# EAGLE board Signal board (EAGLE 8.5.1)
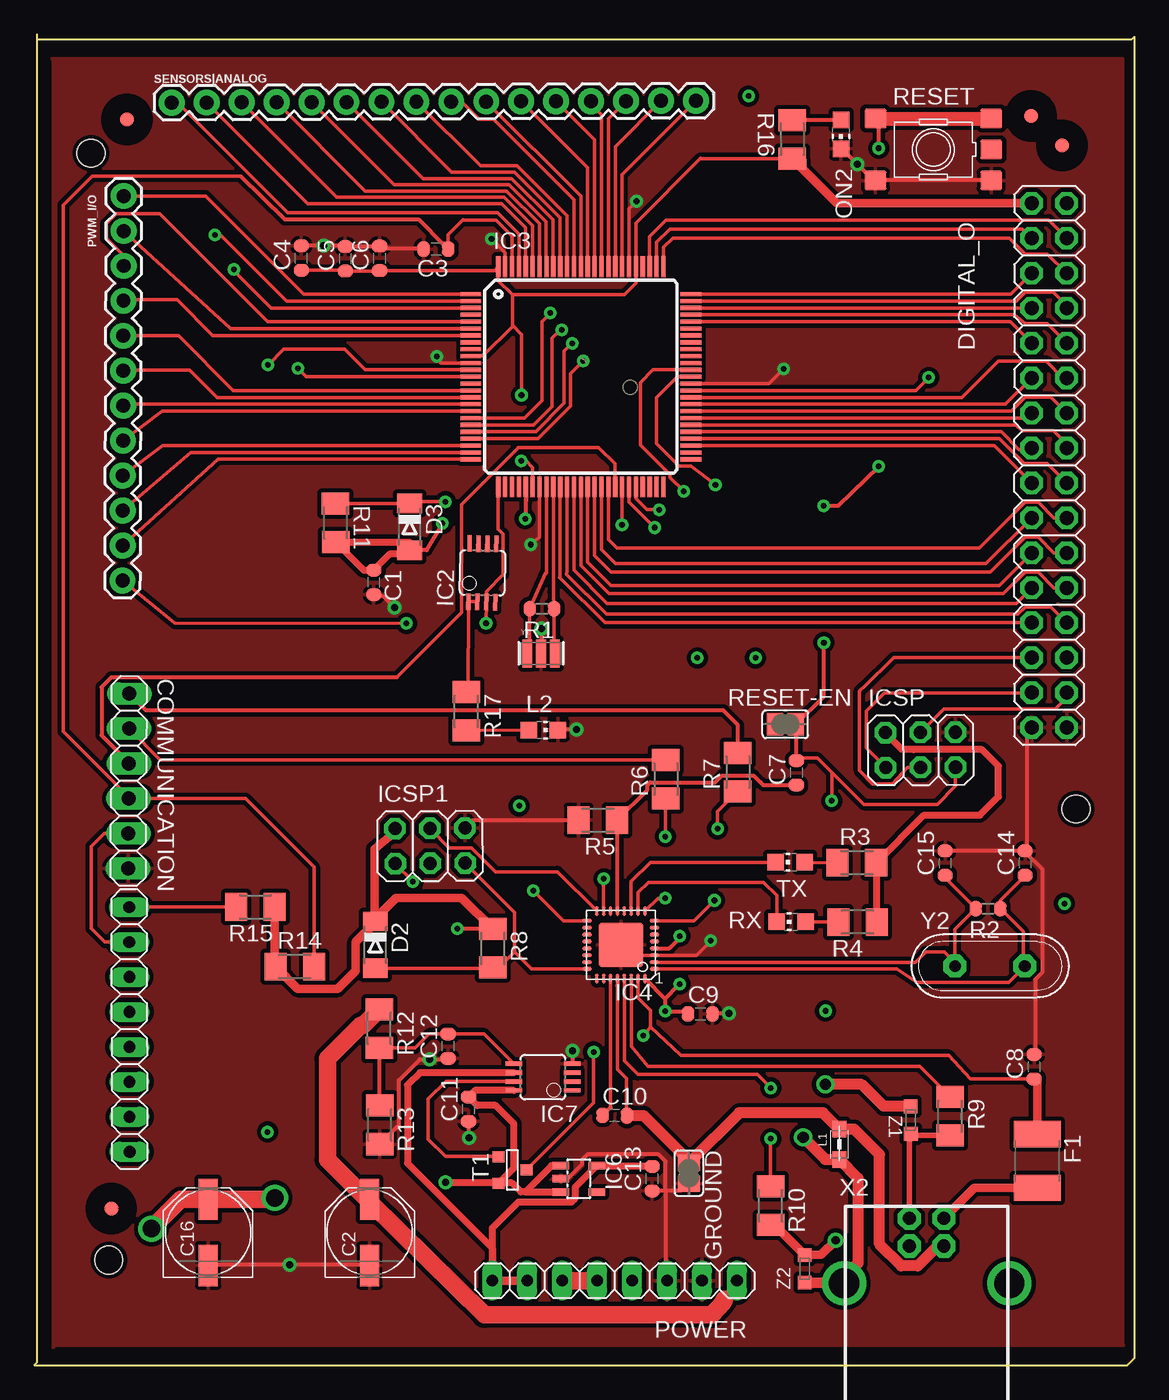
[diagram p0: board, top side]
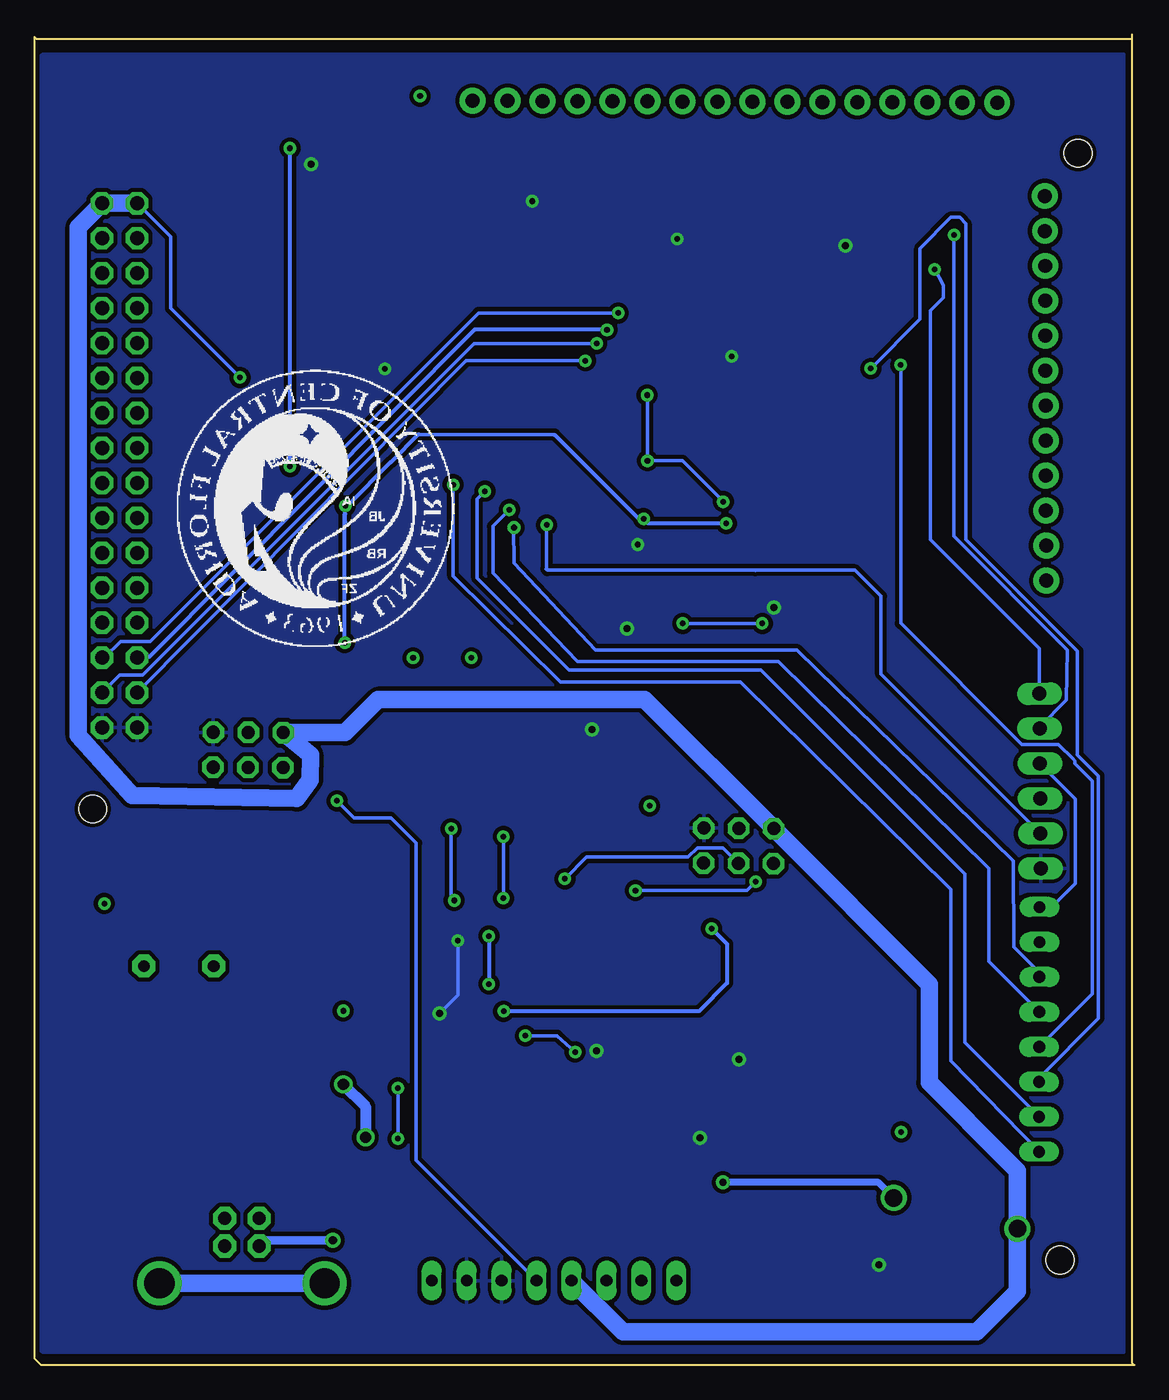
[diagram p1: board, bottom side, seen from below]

Size 79.92 x 96.68 mm. Coordinates in mm from the lower left corner, seen from the top.
Outline: 0.17,96.34 79.75,96.34 79.92,96.51 79.92,0.51 79.41,0 0,0 0.17,0.17 0.17,96.68
Copper layers (1*16): Top 0.035mm / dielectric 1.5mm / Bottom 0.035mm
Design rules "SparkFun *": minimum track width 8mil, minimum drill 8mil, track to track 8mil, track to pad 8mil, pad to pad 8mil, via to via 8mil, smd to smd 8mil, copper to edge 8mil, drill to drill 8mil, minimum pad ring 12mil, minimum via ring 10mil, stop-mask expansion 4mil, vias tented up to drill 20mil, thermal gap 10mil
Net classes: 0 default: width 0.203 mm, drill 0.406 mm, clearance 0.203 mm; 1 power: width 0.61 mm, drill 0.406 mm, clearance 0.203 mm; 2 gnd: width 0.305 mm, drill 0.406 mm, clearance 0.203 mm; 3 power usb: width 0.508 mm, drill 0.406 mm, clearance 0.203 mm
Holes 2.03 mm at 5.4,7.64 75.68,40.4 4.1,88.05

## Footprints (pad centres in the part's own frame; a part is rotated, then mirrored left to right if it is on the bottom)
C0603-ROUND = smd 0.898 x 1.1: 1 -0.889,0; 2 0.889,0
PANASONIC_D = smd 3 x 1.4: + 2.4,0; - -2.4,0
1X08 = drill 0.85 pad 1.422 long: 1 -8.89,0; 2 -6.35,0; 3 -3.81,0; 4 -1.27,0; 5 1.27,0; 6 3.81,0; 7 6.35,0; 8 8.89,0
MINIMELF = smd 1.4 x 1.8: A 1.7,0; C -1.7,0
2X16 = drill 1.016 octagon: 1 -19.05,-1.27; 2 -19.05,1.27; 3 -16.51,-1.27; 4 -16.51,1.27; 5 -13.97,-1.27; 6 -13.97,1.27; 7 -11.43,-1.27; 8 -11.43,1.27; 9 -8.89,-1.27; 10 -8.89,1.27; 11 -6.35,-1.27; 12 -6.35,1.27; 13 -3.81,-1.27; 14 -3.81,1.27; 15 -1.27,-1.27; 16 -1.27,1.27; 17 1.27,-1.27; 18 1.27,1.27; 19 3.81,-1.27; 20 3.81,1.27; 21 6.35,-1.27; 22 6.35,1.27; 23 8.89,-1.27; 24 8.89,1.27; 25 11.43,-1.27; 26 11.43,1.27; 27 13.97,-1.27; 28 13.97,1.27; 29 16.51,-1.27; 30 16.51,1.27; 31 19.05,-1.27; 32 19.05,1.27
L1812 = smd 1.9 x 3.4: 1 -1.95,0; 2 1.95,0
FIDUCIA-MOUNT = smd 1.016 x 1.016: P$1 0,0
SJ = smd 1.168 x 1.6: 1 -0.762,0; 2 0.762,0
MSOP08 = smd 0.3 x 1.2: 1 -0.976,-2.113; 2 -0.326,-2.113; 3 0.324,-2.113; 4 0.974,-2.113; 5 0.974,2.112; 6 0.324,2.112; 7 -0.326,2.112; 8 -0.976,2.112
TQFP100 = smd 1.5 x 0.3: 1 -8,6; 2 -8,5.5; 3 -8,5; 4 -8,4.5; 5 -8,4; 6 -8,3.5; 7 -8,3; 8 -8,2.5; 9 -8,2; 10 -8,1.5; 11 -8,1; 12 -8,0.5; 13 -8,0; 14 -8,-0.5; 15 -8,-1; 16 -8,-1.5; 17 -8,-2; 18 -8,-2.5; 19 -8,-3; 20 -8,-3.5; 21 -8,-4; 22 -8,-4.5; 23 -8,-5; 24 -8,-5.5; 25 -8,-6; 51 8,-6; 52 8,-5.5; 53 8,-5; 54 8,-4.5; 55 8,-4; 56 8,-3.5; 57 8,-3; 58 8,-2.5; 59 8,-2; 60 8,-1.5; 61 8,-1; 62 8,-0.5; 63 8,0; 64 8,0.5; 65 8,1; 66 8,1.5; 67 8,2; 68 8,2.5; 69 8,3; 70 8,3.5; 71 8,4; 72 8,4.5; 73 8,5; 74 8,5.5; 75 8,6 | smd 0.3 x 1.5: 26 -6,-8; 27 -5.5,-8; 28 -5,-8; 29 -4.5,-8; 30 -4,-8; 31 -3.5,-8; 32 -3,-8; 33 -2.5,-8; 34 -2,-8; 35 -1.5,-8; 36 -1,-8; 37 -0.5,-8; 38 0,-8; 39 0.5,-8; 40 1,-8; 41 1.5,-8; 42 2,-8; 43 2.5,-8; 44 3,-8; 45 3.5,-8; 46 4,-8; 47 4.5,-8; 48 5,-8; 49 5.5,-8; 50 6,-8; 76 6,8; 77 5.5,8; 78 5,8; 79 4.5,8; 80 4,8; 81 3.5,8; 82 3,8; 83 2.5,8; 84 2,8; 85 1.5,8; 86 1,8; 87 0.5,8; 88 0,8; 89 -0.5,8; 90 -1,8; 91 -1.5,8; 92 -2,8; 93 -2.5,8; 94 -3,8; 95 -3.5,8; 96 -4,8; 97 -4.5,8; 98 -5,8; 99 -5.5,8; 100 -6,8
MLF32 = smd 0.7 x 0.28: 1 -2.45,1.75; 2 -2.45,1.25; 3 -2.45,0.75; 4 -2.45,0.25; 5 -2.45,-0.25; 6 -2.45,-0.75; 7 -2.45,-1.25; 8 -2.45,-1.75; 17 2.45,-1.75; 18 2.45,-1.25; 19 2.45,-0.75; 20 2.45,-0.25; 21 2.45,0.25; 22 2.45,0.75; 23 2.45,1.25; 24 2.45,1.75 | smd 0.28 x 0.7: 9 -1.75,-2.45; 10 -1.25,-2.45; 11 -0.75,-2.45; 12 -0.25,-2.45; 13 0.25,-2.45; 14 0.75,-2.45; 15 1.25,-2.45; 16 1.75,-2.45; 25 1.75,2.45; 26 1.25,2.45; 27 0.75,2.45; 28 0.25,2.45; 29 -0.25,2.45; 30 -0.75,2.45; 31 -1.25,2.45; 32 -1.75,2.45 | smd 3.254 x 3.254: 33 0,0
SOT23-DBV = smd 0.55 x 1.2: 1 -0.95,-1.3; 2 0,-1.3; 3 0.95,-1.3; 4 0.95,1.3; 5 -0.95,1.3
2X03 = drill 0.95 pad 1.55 octagon: 1 -2.54,-1.27; 2 -2.54,1.27; 3 0,-1.27; 4 0,1.27; 5 2.54,-1.27; 6 2.54,1.27
0805 = smd 1.2 x 1: 1 -1.1,0; 2 1.1,0
CHIP-LED0805 = smd 1.2 x 1.2: A 0,-1.05; C 0,1.05
1X12 = drill 1.016 pad 1.88: 1 0,0; 2 2.54,0; 3 5.08,0; 4 7.62,0; 5 10.16,0; 6 12.7,0; 7 15.24,0; 8 17.78,0; 9 20.32,0; 10 22.86,0; 11 25.4,0; 12 27.94,0
R0603-ROUND = smd 0.898 x 1.1: 1 -0.889,0; 2 0.889,0
M1206 = smd 1.6 x 2: 1 -1.4,0; 2 1.4,0
TS42 = smd 1.6 x 1.4: 1 -4.2,2.25; 2 4.2,2.25; 3 -4.2,-2.25; 4 4.2,-2.25; 5 -4.2,0
1X16 = drill 1.016 pad 1.88: 1 0,0; 2 2.54,0; 3 5.08,0; 4 7.62,0; 5 10.16,0; 6 12.7,0; 7 15.24,0; 8 17.78,0; 9 20.32,0; 10 22.86,0; 11 25.4,0; 12 27.94,0; 13 30.48,0; 14 33.02,0; 15 35.56,0; 16 38.1,0
SOT-23 = smd 0.787 x 0.889: 1 0.025,-1.016; 2 -0.94,1.016; 3 0.991,1.016
PN61729 = drill 0.95 pad 1.676 octagon: 1 1.25,4.71; 2 -1.25,4.71; 3 -1.25,2.71; 4 1.25,2.71 | drill 2.2: P$1 -6,0; P$2 6,0
RESONATOR = smd 0.7 x 2: 1 -1,0; 2 0,0; 3 1,0
QS = drill 0.85 pad 1.676 octagon: 1 -2.54,0; 2 2.54,0
CT/CN0603 = smd 1 x 1: 1 -1,0; 2 1,0
1X06 = drill 1.016 long: 1 -6.35,0; 2 -3.81,0; 3 -1.27,0; 4 1.27,0; 5 3.81,0; 6 6.35,0

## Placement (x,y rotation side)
C1  22p  [C0603-ROUND]  24.66,56.87 270 top
C2  [PANASONIC_D]  24.36,9.64 90 top
C3  100n  [C0603-ROUND]  29.18,81.08 180 top
C4  100n  [C0603-ROUND]  19.39,80.43 90 top
C5  100n  [C0603-ROUND]  22.59,80.38 90 top
C6  100n  [C0603-ROUND]  25.09,80.42 90 top
C7  100n  [C0603-ROUND]  55.37,43.03 90 top
C8  100n  [C0603-ROUND]  72.64,21.67 90 top
C9  100n  [C0603-ROUND]  48.38,25.51 0 top
C10  1u  [C0603-ROUND]  42.17,18.14 0 top
C11  100n  [C0603-ROUND]  31.55,18.6 90 top
C12  100n  [C0603-ROUND]  30.06,23.17 90 top
C13  1u  [C0603-ROUND]  44.88,13.54 90 top
C14  22p  [C0603-ROUND]  71.99,36.48 90 top
C15  22p  [C0603-ROUND]  66.17,36.47 90 top
C16  [PANASONIC_D]  12.62,9.64 90 top
COMMUNICATION  [1X08]  6.9,24.39 270.1 top
D2  CD1206-S01575  [MINIMELF]  24.78,30.53 270 top
D3  CD1206-S01575  [MINIMELF]  27.27,60.9 270 top
DIGITAL_O  [2X16]  73.73,65.36 270 top
F1  MF-MSMF050-2 500mA  [L1812]  72.88,14.83 270 top
FD1  FIDUCIALMOUNT  [FIDUCIA-MOUNT]  6.74,90.51 0 top
FD2  FIDUCIALMOUNT  [FIDUCIA-MOUNT]  72.41,90.77 0 top
FD3  FIDUCIALMOUNT  [FIDUCIA-MOUNT]  5.58,11.39 0 top
FD4  FIDUCIALMOUNT  [FIDUCIA-MOUNT]  74.65,88.61 0 top
GROUND  [SJ]  47.55,13.94 270 top
IC2  LMV358IDGKR  [MSOP08]  32.55,57.57 358.9 top
IC3  ATMEGA2560-16AU  [TQFP100]  39.7,71.81 0 top
IC4  ATMEGA16U2-MU  [MLF32]  42.61,30.53 180 top
IC6  LP2985-33DBVR  [SOT23-DBV]  39.55,13.54 270 top
IC7  LMV358IDGKR  [MSOP08]  36.95,20.92 90 top
ICSP  [2X03]  64.39,44.69 0.3 top
ICSP1  [2X03]  28.75,37.72 0.4 top
L1  BLM21  [0805]  58.49,16.04 270 top
L2  YELLOW  [CHIP-LED0805]  36.98,46.14 270 top
ON2  GREEN  [CHIP-LED0805]  58.6,89.41 180 top
POWER  [1X08]  42.16,6.14 0 top
PWM_I/O  [1X12]  6.5,84.94 269.8 top
R1  1M  [R0603-ROUND]  36.88,54.94 180 top
R2  1M  [R0603-ROUND]  69.28,33.16 180 top
R3  1k  [M1206]  59.76,36.49 0 top
R4  1k  [M1206]  59.81,32.19 0 top
R5  1k  [M1206]  40.93,39.6 180 top
R6  1k  [M1206]  45.88,42.58 90 top
R7  1k  [M1206]  51.11,43.08 90 top
R8  10k  [M1206]  33.31,30.28 270 top
R9  22R  [M1206]  66.53,18.08 270 top
R10  22R  [M1206]  53.48,11.58 270 top
R11  10k  [M1206]  21.88,61.19 270.4 top
R12  10k  [M1206]  25.06,24.45 270 top
R13  10k  [M1206]  25.09,17.46 270 top
R14  10k  [M1206]  18.91,28.95 0 top
R15  10k  [M1206]  16.06,33.29 180 top
R16  1k  [M1206]  55.07,89.06 90.3 top
R17  1k  [M1206]  31.38,47.49 270 top
RESET  TS42031-160R-TR-7260  [TS42]  65.32,88.32 180 top
RESET-EN  [SJ]  54.56,46.56 0 top
RX  YELLOW  [CHIP-LED0805]  54.99,32.21 90 top
SENSORS|ANALOG  [1X16]  9.97,91.72 0.2 top
T1  FDN340P  [SOT-23]  34.74,14.15 90 top
TX  YELLOW  [CHIP-LED0805]  54.9,36.53 90 top
X2  USB-B_TH  [PN61729]  64.83,5.94 0 top
Y1  CSTCE16M0V53-R0 16MHZ  [RESONATOR]  36.81,51.7 0 top
Y2  16MHz  [QS]  69.43,28.99 0 top
Z1  CG0603MLC-05E  [CT/CN0603]  63.67,17.8 270.5 top
Z2  CG0603MLC-05E  [CT/CN0603]  55.96,7 90 top
|  [1X06]  6.85,42.43 269.6 top

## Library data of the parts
C1 C3-C15 COMMUNICATION FD1-FD4 IC3 IC4 IC6 ICSP ICSP1 POWER R1 R2 RESET X2 Y1 Y2 = SmartPrj
C2 C16 = rcl; SPICEPREFIX: C
D2 D3 = diode
DIGITAL_O | = pinhead
F1 = rcl
GROUND RESET-EN = jumper
IC2 IC7 = linear
L1 = wuerth-elektronik
L2 ON2 RX TX = led
PWM_I/O SENSORS|ANALOG = SparkFun-Connectors
R3-R17 = rcl; SPICEPREFIX: R
T1 = zetex; OC_FARNELL: unknown; OC_NEWARK: unknown
Z1 Z2 = varistor

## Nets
5-GND: RESET.5
+3V3 [power]: C13.2 IC6.5 IC7.6 POWER.1 POWER.2
+5V [power usb]: C4.1 C5.1 C6.1 C9.1 C11.2 C16.+ D2.C D3.C DIGITAL_O.1 DIGITAL_O.2 IC3.10 IC3.31 IC3.61 IC3.80 IC3.100 IC4.4 IC4.32 IC6.1 IC6.3 IC7.8 ICSP1.2 ICSP.2 POWER.3 POWER.4 R3.2 R4.2 R8.1 R11.1 R14.1 R15.1 R16.1 T1.2
ADC0: IC3.97 SENSORS|ANALOG.1
ADC1: IC3.96 SENSORS|ANALOG.2
ADC2: IC3.95 SENSORS|ANALOG.3
ADC3: IC3.94 SENSORS|ANALOG.4
ADC4: IC3.93 SENSORS|ANALOG.5
ADC5: IC3.92 SENSORS|ANALOG.6
ADC6: IC3.91 SENSORS|ANALOG.7
ADC7: IC3.90 SENSORS|ANALOG.8
ADC8: IC3.89 SENSORS|ANALOG.9
ADC9: IC3.88 SENSORS|ANALOG.10
ADC10: IC3.87 SENSORS|ANALOG.11
ADC11: IC3.86 SENSORS|ANALOG.12
ADC12: IC3.85 SENSORS|ANALOG.13
ADC13: IC3.84 SENSORS|ANALOG.14
ADC14: IC3.83 SENSORS|ANALOG.15
ADC15: IC3.82 SENSORS|ANALOG.16
AREF: C3.1 IC3.98 R14.2 |.4
CMP: C12.2 IC7.5 R12.2 R13.1
D+: R10.2 X2.3 Z2.2
D-: R9.2 X2.2 Z1.2
DTR: C7.1 IC4.13 R5.1
GATE_CMD: IC7.7 T1.3
GND [gnd]: C1.2 C2.- C3.2 C4.2 C5.2 C6.2 C8.2 C9.2 C11.1 C12.1 C13.1 C14.2 C15.2 C16.- DIGITAL_O.31 DIGITAL_O.32 GROUND.2 IC3.11 IC3.32 IC3.62 IC3.81 IC3.99 IC4.3 IC4.33 IC6.2 IC7.4 ICSP1.6 ICSP.6 L2.C ON2.C POWER.6 POWER.7 R5.2 R13.2 RESET.1 RESET.2 Y1.2 |.6
L13: IC2.1 IC2.2 R17.1
M8RXD: IC4.9 R6.1
M8TXD: IC4.8 R7.1
MISO2: IC4.17 ICSP1.1
MOSI2: IC4.16 ICSP1.4
N$10: L2.A R17.2
N$11: ON2.A R16.2
N$54: R4.1 RX.A
N$55: R3.1 TX.A
PA0: DIGITAL_O.4 IC3.78
PA1: DIGITAL_O.3 IC3.77
PA2: DIGITAL_O.6 IC3.76
PA3: DIGITAL_O.5 IC3.75
PA4: DIGITAL_O.8 IC3.74
PA5: DIGITAL_O.7 IC3.73
PA6: DIGITAL_O.10 IC3.72
PA7: DIGITAL_O.9 IC3.71
PB0: DIGITAL_O.28 IC3.19
PB1: DIGITAL_O.27 IC3.20 ICSP.3
PB2: DIGITAL_O.30 IC3.21 ICSP.4
PB3: DIGITAL_O.29 IC3.22 ICSP.1
PB4: IC3.23 PWM_I/O.9
PB5: IC3.24 PWM_I/O.10
PB6: IC3.25 PWM_I/O.11
PB7: IC2.3 IC3.26 PWM_I/O.12
PC0: DIGITAL_O.17 IC3.53
PC1: DIGITAL_O.18 IC3.54
PC2: DIGITAL_O.15 IC3.55
PC3: DIGITAL_O.16 IC3.56
PC4: DIGITAL_O.13 IC3.57
PC5: DIGITAL_O.14 IC3.58
PC6: DIGITAL_O.11 IC3.59
PC7: DIGITAL_O.12 IC3.60
PE0: IC3.2 R6.2 |.2
PE1: IC3.3 R7.2 |.1
PE3: IC3.5 PWM_I/O.3
PE4: IC3.6 PWM_I/O.2
PE5: IC3.7 PWM_I/O.4
PG5: IC3.1 PWM_I/O.1
PH3: IC3.15 PWM_I/O.5
PH4: IC3.16 PWM_I/O.6
PH5: IC3.17 PWM_I/O.7
PH6: IC3.18 PWM_I/O.8
PL0: DIGITAL_O.25 IC3.35
PL1: DIGITAL_O.26 IC3.36
PL2: DIGITAL_O.23 IC3.37
PL3: DIGITAL_O.24 IC3.38
PL4: DIGITAL_O.21 IC3.39
PL5: DIGITAL_O.22 IC3.40
PL6: DIGITAL_O.19 IC3.41
PL7: DIGITAL_O.20 IC3.42
RD+: IC4.29 R10.1
RD-: IC4.30 R9.1
RESET: C1.1 C7.2 D3.A IC3.30 ICSP.5 POWER.5 R11.2 RESET-EN.1 RESET-EN.2 RESET.3 RESET.4
RESET2: D2.A IC4.24 ICSP1.5 R8.2
RXD1: COMMUNICATION.3 IC3.45
RXD2: COMMUNICATION.5 IC3.12
RXD3: COMMUNICATION.8 IC3.63
RXL: IC4.10 RX.C
SCK2: IC4.15 ICSP1.3
SCL: COMMUNICATION.1 IC3.43 R15.2 |.3
SDA: COMMUNICATION.2 IC3.44 |.5
TXD1: COMMUNICATION.4 IC3.46
TXD2: COMMUNICATION.6 IC3.13
TXD3: COMMUNICATION.7 IC3.64
TXL: IC4.11 TX.C
UGND [gnd]: C10.2 GROUND.1 IC4.28 L1.1 X2.4
USBVCC [power usb]: C8.1 F1.1 IC4.31 T1.1
USHIELD [gnd]: L1.2 X2.P$1 X2.P$2 Z1.1 Z2.1
V+: IC2.8
V-: IC2.4
VIN [power]: C2.+ R12.1
VUCAP: C10.1 IC4.27
XT1: C14.1 IC4.1 R2.1 Y2.2
XT2: C15.1 IC4.2 R2.2 Y2.1
XTAL1: IC3.34 R1.1 Y1.3
XTAL2: IC3.33 R1.2 Y1.1
XVCC [power usb]: F1.2 X2.1

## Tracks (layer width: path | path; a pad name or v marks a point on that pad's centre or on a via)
+3V3
  Top 0.508: C13.2 40.9,14.43 IC6.5 39.3,12.94 39.3,12.12 39.03,11.85 35.16,11.85 33.27,9.96 POWER.1 33.27,8.49 27.1,14.66 27.1,20.34 28,21.25 IC7.6
  Top 0.61: POWER.1 POWER.2
+5V  (via drill 0.41, 0.51, 1.27)
  Top 0.254: 25.08,79.52 C6.1 | C4.1 22.59,79.54 | C5.1 25.05,79.49 C6.1 | R16.1 48.43,87.66 48.41,87.68 43.7,82.98 IC3.80 43.7,78.6 42.87,77.77 34.72,77.77 | IC3.61 64.03,70.81 v64.98,71.76 | v35.37,65.71 35.71,65.71 36.2,65.21 IC3.31 | 34.72,77.77 33.7,78.79 IC3.100 33.51,79.53 C6.1 | IC3.10 31.72,73.33 32.59,73.33 34.72,75.46 34.72,75.55 | 34.72,75.55 34.72,77.77 | v35.4,70.47 35.4,74.87 34.72,75.55 | v29.86,62.73 27.14,62.73 27.02,62.6 D3.C 22.99,62.6 R11.1
  Top 0.305: R8.1 30.76,31.68 v30.72,31.72 | C9.1 47.3,25.71 v45.82,25.71 45.82,26.62 | IC4.32 45.82,26.62 | 45.82,26.62 46.88,27.68 v46.89,27.68 | IC4.4 46.13,30.28 46.9,31.05 v46.9,31.17
  Top 0.508: R4.2 61.62,31.77 61.62,31.56 61.16,32.02 R3.2 64.63,39.96 68.7,39.96 70.05,41.31 70.05,43.52 68.85,44.72 63.87,44.72 63.87,44.73 63.03,44.73 61.84,45.91 ICSP.2 | 34.01,13.22 34.7,13.22 35.34,12.59 35.67,12.59 | 34.01,13.22 33.73,13.22 T1.2 34.84,14.33 34.84,17.54 33.52,18.87 32.16,18.87 C11.2 32.01,19.95 IC7.8 | 35.67,12.59 IC6.3 | v29.89,13.28 33.97,13.27 34.01,13.22 | IC6.1 37.57,14.49 35.67,12.59
  Top 0.61: ICSP1.2 26.19,38.75 24.7,37.49 24.71,32.32 | D2.C 24.71,32.32 | 22.59,79.54 C5.1 | DIGITAL_O.1 58.32,84.41 R16.1 | 24.71,32.32 24.71,32.39 26.28,33.96 31.04,33.96 R8.1 | 24.71,32.32 24.71,32.1 23.35,30.74 23.35,28.64 22.04,27.34 19.12,27.34 R14.1 17.46,29.01 R15.1
  Top 1.27: POWER.3 POWER.4 | v8.5,9.9 10.64,12.04 C16.+ 17.36,12.04 v17.47,12.15
  Bottom 0.254: 72.31,84.41 DIGITAL_O.2 | v64.98,71.76 70.02,76.79 70.02,81.97 DIGITAL_O.1 | v35.4,70.47 35.37,70.45 v35.37,65.71 32.82,65.71 29.86,62.75 v29.86,62.73
  Bottom 0.305: v30.72,31.72 29.59,30.6 29.59,27.75 31.64,25.71 v45.82,25.71 | v46.9,31.17 v46.9,27.69 v46.89,27.68
  Bottom 0.508: v17.47,12.15 18.59,13.27 v29.89,13.28
  Bottom 1.27: 76.73,82.62 76.73,45.74 72.82,41.39 60.85,41.17 59.87,42.52 59.86,44.34 ICSP.2 57.34,45.95 54.94,48.35 35.58,48.35 ICSP1.2 14.89,27.67 14.89,20.53 9.22,14.85 8.5,14.13 v8.5,9.9 8.5,5.36 11.45,2.41 37.16,2.41 POWER.4 | 76.73,82.62 76.61,82.74 | 76.73,82.62 76.73,82.68 DIGITAL_O.2 DIGITAL_O.1
ADC0
  Top 0.254: IC3.97 35.2,82.15 35.21,82.16 33.64,83.74 18.39,83.73 10.35,91.78 SENSORS|ANALOG.1
ADC1
  Top 0.254: IC3.96 35.68,79.83 35.68,82.63 33.93,84.38 19.86,84.38 SENSORS|ANALOG.2
ADC2
  Top 0.254: IC3.95 36.18,79.83 36.18,82.77 34.12,84.84 21.95,84.84 SENSORS|ANALOG.3
ADC3
  Top 0.254: IC3.94 36.68,79.83 36.68,82.92 34.31,85.3 24.04,85.3 SENSORS|ANALOG.4
ADC4
  Top 0.254: IC3.93 37.18,79.83 37.18,83.07 34.49,85.76 26.13,85.76 SENSORS|ANALOG.5
ADC5
  Top 0.254: IC3.92 37.68,79.83 37.68,83.21 34.68,86.21 28.22,86.21 SENSORS|ANALOG.6
ADC6
  Top 0.254: IC3.91 38.18,79.83 38.18,83.36 34.87,86.67 30.32,86.67 SENSORS|ANALOG.7
ADC7
  Top 0.254: IC3.90 38.68,79.83 38.68,83.51 35.06,87.13 32.41,87.13 SENSORS|ANALOG.8
ADC8
  Top 0.254: SENSORS|ANALOG.9 31.04,91.8 32.3,90.53 33.36,90.53 39.2,84.68 IC3.89
ADC9
  Top 0.254: SENSORS|ANALOG.10 39.7,84.93 IC3.88
ADC10
  Top 0.254: SENSORS|ANALOG.11 40.2,86.98 IC3.87
ADC11
  Top 0.254: SENSORS|ANALOG.12 40.7,89.03 IC3.86
ADC12
  Top 0.254: IC3.85 41.2,90.85 40.45,91.6 SENSORS|ANALOG.13
ADC13
  Top 0.254: IC3.84 41.7,90.55 SENSORS|ANALOG.14
ADC14
  Top 0.254: IC3.83 42.2,88.52 SENSORS|ANALOG.15
ADC15
  Top 0.254: IC3.82 42.7,86.49 SENSORS|ANALOG.16
AREF
  Top 0.254: IC3.98 34.7,82.03 33.54,83.19 31.15,83.19 31.14,83.2 30.06,82.13 C3.1 | 30.36,81.37 30.24,81.25 | |.4 6.96,41.16 | 6.96,41.16 15.34,41.16 20.31,36.19 R14.2 | 15,86.37 4.18,86.37 2.1,84.29 2.1,46.03 6.96,41.16
  Top 0.305: 29.74,81.5 29.74,81.4 | 29.74,81.4 C3.1 30.24,81.25 30.37,81.38 | 29.74,81.4 27.89,83.25 18.19,83.25 15,86.37 | 6.46,41.16 |.4
CMP
  Top 0.254: IC7.5 32.68,24.06 C12.2 28.68,24.06 27.65,23.03 25.1,23.03 25.06,22.99
  Top 0.305: R12.2 25.06,22.99 25.06,19.19 R13.1
D+  (via drill 0.61)
  Top 0.61: v58.23,9.07 57.16,8 Z2.2 53.78,10.18 R10.2
  Bottom 0.61: v58.23,9.07 63.17,9.07 X2.3
D-
  Top 0.203: Z1.2 63.73,16.81 63.58,16.8
  Top 0.406: X2.2 63.58,16.8 Z1.2 | Z1.2 | Z1.2 63.68,16.68 R9.2
DTR
  Top 0.305: IC4.13 42.36,39.6 R5.1 44.53,41.79 44.53,42.13 44.74,42.34 49.46,42.34 49.97,42.84 52.26,42.84 52.76,42.34 52.95,42.14 C7.1
GATE_CMD
  Top 0.254: 33.49,20.62 33.68,20.62 | 33.68,20.62 IC7.7 | 33.69,15.21 T1.3 33.72,15.17 33.7,15.19 33.67,15.16 29.87,15.16 28.61,16.42 28.61,19.33 29.9,20.62 33.68,20.62
GND  (via drill 0.41, 0.51)
  Top 0.254: IC4.33 43.36,29.78 IC4.3 48.1,29.78 v49.15,30.82 | IC3.32 36.7,60.16 v36.07,59.61 | IC3.11 29.54,72.81 v29.25,73.27 | IC3.99 34.2,80.84 v33.21,81.83 | IC3.81 43.2,84.02 v43.74,84.56 | IC3.62 53.38,71.31 v54.45,72.38
  Top 0.305: 48.63,5.9 POWER.7 | C15.2 66.21,37.35 71.9,37.35 C14.2 | C8.2 72.71,22.62 72.71,28.01 73.22,28.51 73.22,36.03 72,37.25 C14.2 | C16.- 12.67,7.28 v18.56,7.28 24.35,7.28 C2.- | ON2.C 58.69,88.36 v59.81,87.24 61.03,86.02 RESET.2 61.23,86.12 69.46,86.12 RESET.1 | C12.1 30.04,22.22 v28.72,22.22 28.01,22.22 26.48,20.69 26.48,17.44 25.16,16.12 R13.2 | 45.89,12.67 47.01,12.67 47.52,13.17 GROUND.2 | 45.89,12.67 45.86,12.67 | 45.86,12.67 44.94,12.67 C13.1 | 45.86,12.67 45.86,14.8 45.35,15.31 40.2,15.31 39.79,14.9 39.79,14.6 38.78,13.58 38.27,13.58 IC6.2 | C4.2 19.47,81.35 v21,81.35 22.52,81.35 C5.2 22.62,81.25 25.06,81.25 C6.2 25.16,81.14 28.21,81.14 C3.2 | v31.56,16.53 31.56,17.64 C11.1 | v50.46,25.57 49.34,25.57 C9.2 | v26.18,55.03 25.37,55.85 C1.2 | v39.08,22.83 39.08,21.91 IC7.4 | v39.39,46.19 38.07,46.19 L2.C | R5.2 39.49,39.59 31.87,39.59 31.36,39.08 ICSP1.6 | v36.85,53.51 36.85,51.78 Y1.2 | 45.89,12.67 45.89,6.16 POWER.6 | C14.2 72.1,37.46 72.1,45.99 72.41,46.29 DIGITAL_O.31
  Bottom 0.254: v50.46,25.57 49.15,26.89 v49.15,30.82
  pour Bottom (isolate 0.305): 0.85,0.93 79.32,0.93 79.41,1.02 79.41,95.16 79.32,95.24 0.76,95.24 0.76,0.93
  pour Top (isolate 0.305): 1.27,94.9 79.07,94.9 79.07,1.52 79.16,1.44 1.52,1.44 1.35,1.27 1.35,94.82
L13
  Top 0.254: R17.1 31.52,48.69 IC2.1 IC2.2
M8RXD  (via drill 0.41)
  Top 0.254: v45.85,38.4 45.85,41.14 R6.1 | IC4.9 45.29,33.91 v45.85,33.91
  Bottom 0.254: v45.85,33.91 v45.85,38.4
M8TXD  (via drill 0.41)
  Top 0.254: IC4.8 47.93,32.28 v49.41,33.76 | v49.64,38.96 49.64,40.21 R7.1
  Bottom 0.254: v49.41,33.76 49.64,33.98 v49.64,38.96
MISO2  (via drill 0.41)
  Top 0.254: IC4.17 38.44,32.28 v36.25,34.48 | v27.5,35.12 26.21,36.41 ICSP1.1
  Bottom 0.254: v36.25,34.48 28.15,34.48 v27.5,35.12
MOSI2
  Top 0.254: 28.77,39.16 ICSP1.4 30.15,37.58 31.76,37.58 33.51,35.83 38,35.83 IC4.16
N$2  (via drill 0.41)
  other vias: 35.22,40.64
N$4  (via drill 0.41)
  other vias: 51.9,92.19
N$5  (via drill 0.41)
  other vias: 57.48,25.74
N$6  (via drill 0.41)
  other vias: 48.17,51.39
N$7  (via drill 0.41)
  other vias: 52.4,51.39
N$8  (via drill 0.41)
  other vias: 16.93,16.93
N$9  (via drill 0.41)
  other vias: 74.84,33.52
N$10
  Top 0.254: R17.2 L2.A
N$11
  Top 0.305: ON2.A R16.2
N$54
  Top 0.254: RX.A R4.1
N$55
  Top 0.254: TX.A R3.1
PA0
  Top 0.254: IC3.78 44.7,81.99 45.9,83.18 73.69,83.18 DIGITAL_O.4
PA1
  Top 0.254: IC3.77 45.2,81.57 46.17,82.54 71.8,82.54 DIGITAL_O.3
PA2
  Top 0.254: IC3.76 45.7,81.21 46.39,81.89 70.83,81.89 71.99,80.73 73.6,80.73 DIGITAL_O.6
PA3
  Top 0.254: IC3.75 70.93,77.81 DIGITAL_O.5
PA4
  Top 0.254: IC3.74 71.36,77.31 71.99,77.94 73.95,77.94 73.99,77.98 75,76.98 DIGITAL_O.8
PA5
  Top 0.254: IC3.73 72.44,76.81 DIGITAL_O.7
PA6
  Top 0.254: IC3.72 71.2,76.31 71.99,75.65 73.6,75.65 DIGITAL_O.10
PA7
  Top 0.254: IC3.71 70.9,75.81 DIGITAL_O.9
PB0  (via drill 0.41)
  Top 0.254: IC3.19 35.62,68.81 36.87,70.06 36.87,75.82 v37.5,76.44
  Bottom 0.254: v37.5,76.44 47.65,76.44 71.51,52.58 73.65,52.58 74.84,51.39 DIGITAL_O.28
PB1  (via drill 0.41)
  Top 0.254: DIGITAL_O.27 62.46,51.39 60.22,49.24 60.09,49.11 59.96,48.98 59.96,48.97 59.95,48.97 59.96,48.82 59.96,43.22 60.9,42.22 62.34,42.22 63.43,43.42 ICSP.3 | IC3.20 36.28,68.31 37.63,69.65 37.63,74.62 38.22,75.22 v38.31,75.22
  Bottom 0.254: 72.59,51.41 72.59,51.47 DIGITAL_O.27
  Bottom 0.305: 72.59,51.47 71.55,51.47 47.93,75.24 38.44,75.24 v38.31,75.22
PB2  (via drill 0.41)
  Top 0.254: 64.44,46.02 ICSP.4 66.09,47.67 74.19,47.67 75,48.48 DIGITAL_O.30 | IC3.21 31.72,67.83 36.45,67.83 38.5,69.88 38.5,73.65 v39.07,74.23
  Bottom 0.254: v39.07,74.23 47.97,74.23 72.07,50.13 73.72,50.13 DIGITAL_O.30
PB3  (via drill 0.41)
  Top 0.254: DIGITAL_O.29 72.47,48.84 61.77,48.84 60.44,47.51 60.44,44.82 ICSP.1 | v39.88,72.96 38.96,72.03 38.96,69.69 36.57,67.31 IC3.22
  Bottom 0.254: v39.88,72.96 48.57,72.96 DIGITAL_O.29
PB4
  Top 0.254: IC3.23 9.31,66.81 PWM_I/O.9
PB5
  Top 0.254: IC3.24 11.34,66.31 PWM_I/O.10
PB6
  Top 0.254: IC3.25 13.37,65.81 PWM_I/O.11
PB7  (via drill 0.41)
  Top 0.254: IC3.26 33.7,60.75 34.06,60.39 34.06,57.43 32.83,56.21 IC2.3 32.81,53.91 v32.81,53.89 | PWM_I/O.12 10.19,53.9 v27.03,53.89
  Bottom 0.254: v27.03,53.89 32.9,53.89 v32.81,53.89
PC0
  Top 0.254: IC3.53 69.74,66.81 DIGITAL_O.17
PC1
  Top 0.254: IC3.54 70.11,67.31 71.93,65.49 73.6,65.49 DIGITAL_O.18
PC2
  Top 0.254: IC3.55 70.25,67.81 71.54,66.52 72.35,66.52 DIGITAL_O.15
PC3
  Top 0.254: IC3.56 71.32,68.31 71.73,67.9 74.02,67.9 75,66.92 DIGITAL_O.16
PC4
  Top 0.254: IC3.57 72.09,68.81 DIGITAL_O.13
PC5
  Top 0.254: IC3.58 70.98,69.31 71.99,70.32 73.86,70.32 DIGITAL_O.14
PC6
  Top 0.254: IC3.59 70.55,69.81 DIGITAL_O.11
PC7
  Top 0.254: IC3.60 67.4,70.31 70.03,72.94 73.51,72.94 74.73,71.71 DIGITAL_O.12
PE0  (via drill 0.41)
  Top 0.254: R6.2 9.13,43.98 |.2 | IC3.2 18.32,77.31 13.5,82.12 v13.1,82.12
  Bottom 0.254: 6.87,46.49 |.2 6.87,46.37 4.93,48.31 4.87,51.96 13.12,60.22 13.12,80.4 | 13.12,81.38 13.12,80.4 | v13.1,82.12 13.1,80.42 13.12,80.4
PE1  (via drill 0.41)
  Top 0.254: 51.18,44.31 R7.2 | IC3.3 17.19,76.81 14.85,79.15 v14.51,79.61
  Top 0.305: R7.2 51.11,46.5 50.05,47.56 8.11,47.56 |.1
  Bottom 0.254: |.1 6.89,52.08 14.81,59.99 14.81,76.6 13.86,77.56 13.86,78.45 v14.51,79.61
PE3
  Top 0.254: IC3.5 31.68,75.83 16.94,75.83 9.1,83.67 7.02,83.67 5.96,83.67 5.21,82.93 5.21,81.87 6.48,80.61 PWM_I/O.3
PE4
  Top 0.254: PWM_I/O.2 14.27,75.31 IC3.6
PE5
  Top 0.254: IC3.7 12.96,74.81 10.37,77.39 7.23,77.39 PWM_I/O.4
PG5
  Top 0.254: IC3.1 19.58,77.81 12.44,84.94 7.19,84.94 PWM_I/O.1
PH3
  Top 0.254: PWM_I/O.5 10.47,74.78 14.44,70.81 IC3.15
PH4
  Top 0.254: IC3.16 13.26,70.31 11.27,72.3 7.21,72.3 PWM_I/O.6
PH5
  Top 0.254: IC3.17 7.24,69.81 PWM_I/O.7
PH6
  Top 0.254: IC3.18 9.27,69.31 PWM_I/O.8
PL0
  Top 0.254: IC3.35 38.2,57.24 38.16,57.2 38.26,57.12 41.44,53.93 DIGITAL_O.25
PL1
  Top 0.254: IC3.36 38.7,57.6 38.66,57.56 38.66,57.44 41.55,54.55 71.46,54.55 71.99,55.08 73.86,55.08 DIGITAL_O.26
PL2
  Top 0.254: IC3.37 39.2,57.76 41.62,55.34 71.33,55.34 DIGITAL_O.23
PL3
  Top 0.254: IC3.38 39.7,58.1 41.76,56.04 70.41,56.04 71.99,57.62 72.93,57.62 74.08,56.47 DIGITAL_O.24
PL4
  Top 0.254: 40.2,63.77 IC3.39 40.2,58.34 41.9,56.65 70.09,56.65 DIGITAL_O.21
PL5
  Top 0.254: IC3.40 40.7,58.82 41.9,57.63 69.46,57.63 71.99,60.16 72.93,60.16 74.08,59.01 DIGITAL_O.22
PL6
  Top 0.254: IC3.41 41.2,59.26 42.23,58.23 69.14,58.23 DIGITAL_O.19
PL7
  Top 0.254: IC3.42 41.7,59.96 42.32,59.35 68.64,59.35 71.99,62.7 72.93,62.7 74.08,61.55 DIGITAL_O.20
RD+  (via drill 0.41)
  Top 0.254: IC4.29 42.86,22.1 43.85,21.11 52.53,21.11 v53.5,20.14 | R10.1 53.48,16.44 v53.5,16.45
  Bottom 0.254: v53.5,16.45 v53.5,20.14
RD-
  Top 0.254: 66.46,19.56 R9.1 64.32,21.7 44.59,21.7 43.39,23.15 43.39,28.05 IC4.30
RESET  (via drill 0.41)
  Top 0.254: 55.37,44.1 56.9,44.1 57.94,43.07 | 57.94,43.07 60.26,40.75 65.61,40.75 66.93,42.07 ICSP.5 | 57.94,43.07 v57.94,41
  Top 0.305: RESET-EN.1 RESET-EN.2 | C7.2 55.37,44.1 55.37,46.56 RESET-EN.2 | v61.34,88.41 61.34,90.57 RESET.4 | 35.7,62.91 35.69,62.89 35.69,62.71 | RESET-EN.2 57.35,48.59 57.35,49.19 57.35,52.47 v57.37,52.49 | v61.34,65.3 58.39,62.42 v57.34,62.42 | 35.69,62.71 35.69,61.53 v35.65,61.49 | IC3.30 35.7,62.72 35.69,62.71 | v29.65,61.16 28.5,59.2 D3.A
  Top 0.508: R11.2 27.28,59.79 27.28,58.96 25.86,58.96 C1.1 23.93,57.76 R11.2
  Top 0.61: 27.28,58.96 D3.A
  Top 1.016: RESET.4 RESET.3
  Bottom 0.254: POWER.5 52.18,14.89 52.18,37.93 54,39.75 56.69,39.75 v57.94,41
  Bottom 0.305: v61.34,65.3 v61.34,88.4 v61.34,88.41 | 57.35,61.24 57.34,61.25 57.34,61.85 | 57.34,61.85 v57.34,62.42 57.21,62.42 54.03,65.6 54.02,65.6 52,67.62 42.13,67.6 36.02,61.49 v35.65,61.49 35.32,61.16 v29.65,61.16 | v57.37,52.49 57.37,61.83 57.34,61.85
RESET2
  Top 0.254: ICSP1.5 34.88,32.88 34.88,30.01 | 34.88,30.01 33.76,28.88 33.5,28.88 | 33.5,28.88 R8.2 | D2.A 33.44,28.83 33.5,28.88 | IC4.24 36.11,28.78 34.88,30.01
RXD1  (via drill 0.41)
  Top 0.254: IC3.45 43.2,62.71 v45.06,60.85
  Bottom 0.254: COMMUNICATION.3 6.9,28.51 8.76,30.38 8.8,36.62 24.53,51.97 39.14,51.97 45.05,58.26 45.09,60.82
  Bottom 0.406: 45.09,60.82 v45.06,60.85
RXD2  (via drill 0.41)
  Top 0.254: IC3.12 24.04,72.31 22.54,73.8 18.12,73.8 v16.98,72.66
  Bottom 0.254: COMMUNICATION.5 3.06,26.97 3.06,42.45 4.32,43.71 4.32,43.89 4.45,44.02 5.52,45.09 8.16,45.09 16.98,53.9 v16.98,72.66
RXD3  (via drill 0.41)
  Top 0.254: 47.68,71.79 47.68,71.83 IC3.63 46.73,71.81 45.21,70.29 45.21,66.93 46.82,65.33 47.71,65.33 v49.48,63.96
  Bottom 0.254: COMMUNICATION.8 13.34,22.12 13.34,34.55 28.6,49.61 41.69,49.61 49.48,57.32 v49.48,63.96
RXL
  Top 0.254: RX.C 53.94,34.12 52.98,35.08 44.62,35.08 43.86,34.32 IC4.10
SCK2  (via drill 0.41)
  Top 0.254: IC4.15 41.36,35.32 v41.37,35.33
  Bottom 0.254: v41.37,35.33 39.79,36.91 32.43,36.91 31.76,37.58 29.89,37.58 ICSP1.3
SCL
  Top 0.254: COMMUNICATION.1 R15.2 | |.3 6.86,43.95 | IC3.43 42.18,63.83 42.18,65.48 41,66.66 35.14,66.66 35.14,66.61 31.04,62.51 31.04,54.68 26.32,49.96
  Top 0.305: 26.32,49.96 5.6,49.96 4.89,49.25 4.89,45.76 6.86,43.79 |.3
  Bottom 0.254: |.3 4.28,41.12 4.28,34.98 5.98,33.28 COMMUNICATION.1
SDA  (via drill 0.41)
  Top 0.254: |.5 5.08,38.62 4.14,37.68 4.14,31.72 5.12,30.74 COMMUNICATION.2 | IC3.44 42.7,61.06 v42.69,61.04
  Bottom 0.254: 27.54,57.75 42.64,57.75 42.7,57.8 | 42.7,57.8 42.74,57.85 | |.5 18.41,50.21 18.41,55.86 20.3,57.75 27.54,57.75 | 27.53,57.74 27.54,57.75 | v42.69,61.04 42.69,57.81 42.7,57.8
TXD1  (via drill 0.41)
  Top 0.254: 43.72,63.79 IC3.46 43.7,62.94 44.5,62.15 v45.4,62.15
  Bottom 0.254: COMMUNICATION.4 10.56,29.32 10.56,36.08 25.87,51.12 40.46,51.12 46.6,57.53 46.6,60.94 v45.4,62.15
TXD2  (via drill 0.41)
  Top 0.254: v19.15,72.4 19.74,71.81 IC3.13
  Bottom 0.254: COMMUNICATION.6 6.91,20.88 2.6,25.19 2.6,42.82 4.13,44.34 4.13,51.87 12.24,59.99 12.24,82.94 12.69,83.38 13.31,83.38 15.57,81.13 15.57,75.98 v19.15,72.4
TXD3  (via drill 0.41)
  Top 0.254: 48.22,72.29 48.24,72.31 IC3.64 44.94,72.31 44.03,71.39 44.03,66.85 46.18,64.69 46.18,64.49 v47.18,63.49
  Bottom 0.254: COMMUNICATION.7 12.32,23.44 12.32,35.69 27.12,50.49 41.07,50.49 47.75,57.17 47.75,62.92 v47.18,63.49
TXL
  Top 0.254: TX.C 44.77,36.53 44.77,36.54 43.36,35.13 IC4.11
UGND
  Top 0.254: C10.2 | 42.36,27.55 42.36,21.5 43.03,20.83 43.03,17.92 43.06,17.9
  Top 0.305: IC4.28 42.36,27.55 42.36,27.57
  Top 0.813: C10.2 42.99,17.92 | 43.06,17.9 C10.2 | X2.4 65.63,8.65 64.18,7.2 62.98,7.2 61.41,8.78 61.41,15.3 59.56,17.14 L1.1 57.29,18.34 51.21,18.34 47.63,14.76 | 47.63,14.76 47.25,14.37 47.23,14.37 47.23,14.39 GROUND.1 | C10.2 44.25,18.14 47.63,14.76
USBVCC  (via drill 0.41)
  Top 0.254: T1.1 40.63,19.05 v40.63,22.74 | v44.25,23.93 44.77,24.57 | 44.77,24.57 44.77,25.76 43.86,26.67 IC4.31 | 44.77,24.57 46.99,22.5 66.43,22.5 67.99,20.78 C8.1
  Top 0.61: F1.1 72.88,20.55 arc90 C8.1
  Bottom 0.254: v40.63,22.74 41.93,23.93 v44.25,23.93
USHIELD  (via drill 0.81)
  Top 0.813: Z2.1 58.49,6.04 | 58.49,6.04 X2.P$1 | Z1.1 61.71,18.8 60.11,20.39 v57.47,20.39 | v55.86,16.55 57.47,14.94 L1.2 59.84,13.59 59.84,7.4 58.49,6.04
  Bottom 0.813: v57.47,20.39 55.86,18.78 v55.86,16.55
  Bottom 1.27: X2.P$1 X2.P$2
VIN
  Top 1.27: 50.15,4.79 50.02,4.53 49.22,3.65 32.7,3.65 24.36,11.86 | 24.36,11.86 C2.+ | R12.1 23.89,24.69 23.71,24.69 21.29,22.27 21.29,14.93 24.36,11.86
VUCAP
  Top 0.254: IC4.27 41.86,18.72
  Top 0.305: 41.86,18.72 C10.1
XT1
  Top 0.254: IC4.1 62.66,28.79 64.11,27.82 70.8,27.82 71.84,28.86 | Y2.2 71.84,28.86 | C14.1 70.17,33.77 R2.1 71.84,31.49 71.84,28.86
XT2
  Top 0.254: IC4.2 45.06,29.27 64,29.27 64.77,30.03 66.11,30.03 66.89,29.26 Y2.1 66.89,31.66 R2.2 66.17,35.38 C15.1
XTAL1
  Top 0.254: IC3.34 37.7,56.15 R1.1 37.77,51.74 Y1.3
XTAL2
  Top 0.254: IC3.33 37.2,60.31 37.21,59.92 37.21,57.54 | 37.21,57.54 37.19,57.52 | 37.21,57.54 37.13,57.54 R1.2 35.99,51.88 Y1.1
XVCC
  Top 0.61: F1.2 68.31,12.88 X2.1

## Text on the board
Name: Rev.A | 5V | 5V | EN1 | DI1 | EN2 | DI2 | EN3 | DI3 | EN4 | DI4 | EN5 | DI5 | EN6 | DI6 | EN7 | DI7 | EN8 | DI8 | DI9 | EN9 | EN10 | DI10 | LED1 | LED3 | LED2 | LED4 | SCK | SS | TX>1 | MISO | MOSI | MOSI | RX<0 | 5V | GND | GND | SCL | MISO | SCK | RESET | AREF | MOSI2 | GND | SDA | 5V | GND | MISO2 | SCK2 | RESET2 | SCL | SDA | RX1 | TX1 | RX2 | TX2 | TX3 | RX3 | 3.3V | 5V | RESET | GND | VIN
